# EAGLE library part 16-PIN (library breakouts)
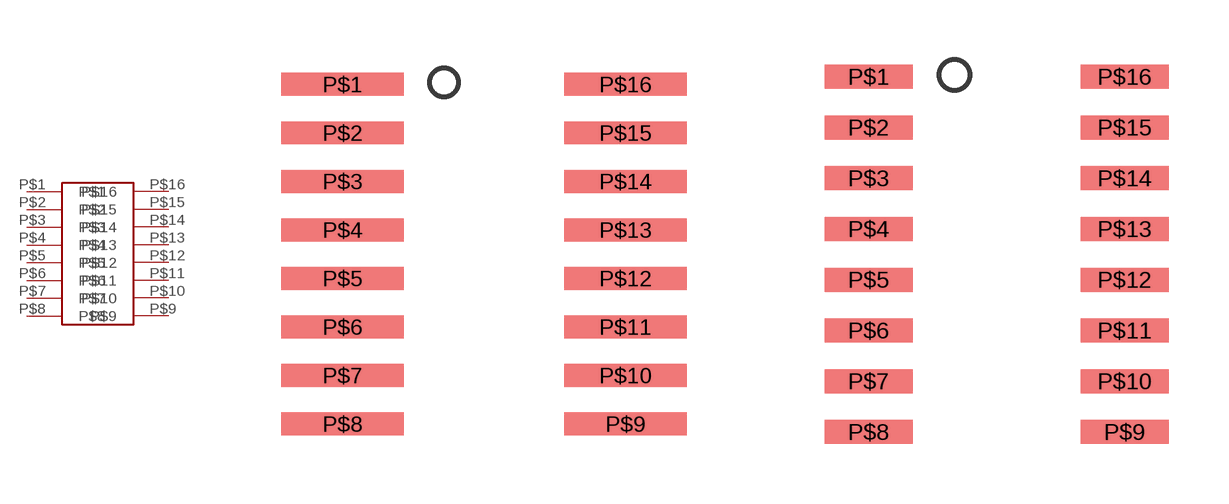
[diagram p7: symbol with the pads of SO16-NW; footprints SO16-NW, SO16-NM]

Designator prefix -

## 16-PINSOIC-NW  [SO16-NW]
P$1  P$1
P$2  P$2
P$3  P$3
P$4  P$4
P$5  P$5
P$6  P$6
P$7  P$7
P$8  P$8
P$9  P$9
P$10  P$10
P$11  P$11
P$12  P$12
P$13  P$13
P$14  P$14
P$15  P$15
P$16  P$16

## 16-PINSOIC-NM  [SO16-NM]
Pads as for SO16-NW

## 16-PINSOIC-M  [SO16-M]
Pads as for SO16-NW

## 16-PINTSSOP-N  [TSSOP16-3.9]
Pads as for SO16-NW

## 16-PINSOIC-N  [SO16-N]
Pads as for SO16-NW

## 16-PINSOIC-MW  [SO16-MW]
Pads as for SO16-NW

## 16-PINSOIC-W  [SO16-W]
Pads as for SO16-NW

## 16-PINTSSOP-W  [TSSOP16-5.3]
Pads as for SO16-NW

## 16-PINTSSOP-NW  [TSSOP16-NW]
Pads as for SO16-NW

## Footprint SO16-NW (pad centres in mm)
smd 3.2 x 0.6: P$1 -3.7,4.445; P$2 -3.7,3.175; P$3 -3.7,1.905; P$4 -3.7,0.635; P$5 -3.7,-0.635; P$6 -3.7,-1.905; P$7 -3.7,-3.175; P$8 -3.7,-4.445; P$9 3.7,-4.445; P$10 3.7,-3.175; P$11 3.7,-1.905; P$12 3.7,-0.635; P$13 3.7,0.635; P$14 3.7,1.905; P$15 3.7,3.175; P$16 3.7,4.445

## Footprint SO16-NM (pad centres in mm)
smd 2.2 x 0.6: P$1 -3.2,4.445; P$2 -3.2,3.175; P$3 -3.2,1.905; P$4 -3.2,0.635; P$5 -3.2,-0.635; P$6 -3.2,-1.905; P$7 -3.2,-3.175; P$8 -3.2,-4.445; P$9 3.2,-4.445; P$10 3.2,-3.175; P$11 3.2,-1.905; P$12 3.2,-0.635; P$13 3.2,0.635; P$14 3.2,1.905; P$15 3.2,3.175; P$16 3.2,4.445

## Footprint SO16-M (pad centres in mm)
smd 1.2 x 0.6: P$1 -3.7,4.445; P$2 -3.7,3.175; P$3 -3.7,1.905; P$4 -3.7,0.635; P$5 -3.7,-0.635; P$6 -3.7,-1.905; P$7 -3.7,-3.175; P$8 -3.7,-4.445; P$9 3.7,-4.445; P$10 3.7,-3.175; P$11 3.7,-1.905; P$12 3.7,-0.635; P$13 3.7,0.635; P$14 3.7,1.905; P$15 3.7,3.175; P$16 3.7,4.445

## Footprint TSSOP16-3.9 (pad centres in mm)
smd 1.4 x 0.35: P$1 -2.65,2.275; P$2 -2.65,1.625; P$3 -2.65,0.975; P$4 -2.65,0.325; P$5 -2.65,-0.325; P$6 -2.65,-0.975; P$7 -2.65,-1.625; P$8 -2.65,-2.275; P$9 2.65,-2.275; P$10 2.65,-1.625; P$11 2.65,-0.975; P$12 2.65,-0.325; P$13 2.65,0.325; P$14 2.65,0.975; P$15 2.65,1.625; P$16 2.65,2.275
